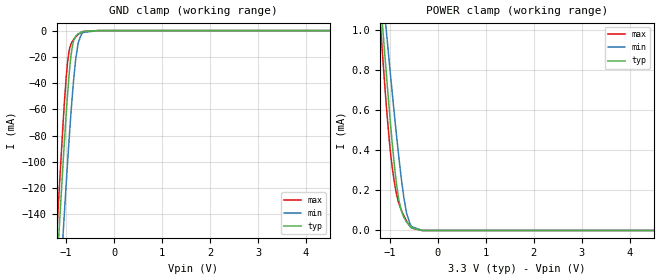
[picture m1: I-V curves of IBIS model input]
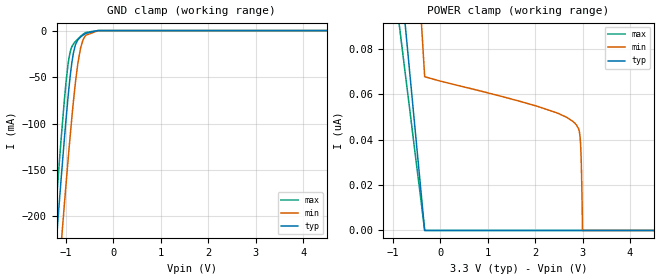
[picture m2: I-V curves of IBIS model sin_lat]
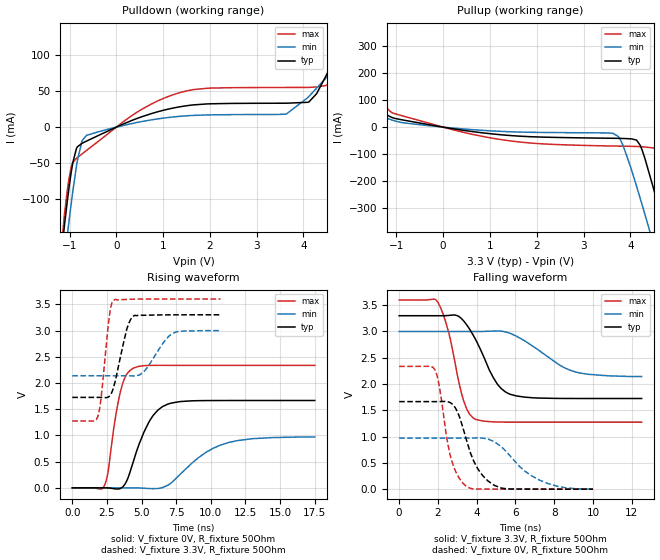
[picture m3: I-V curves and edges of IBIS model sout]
|Texas Instruments Incorporated
| 48 channels constant current LED driver with global brightness control,
| LED open-short detection and power save mode
| Marketing part#   Digital Voltage Range   Package-type   #pins
| TLC5954RTQR   3.0V-3.6V   QFN   56
| TLC5954RTQT   3.0V-3.6V   QFN   56
[IBIS Ver]   4.1
[File name]   tlc5954.ibs
[File Rev]   1.0
[Date]   2/19/2014
[Source]
| Texas Instruments Incorporated.
| Analog-eLab Design Center, HPA
| 12500 TI Blvd
| Dallas, TX -75243
[Notes]   Revision History:
| Rev 1.0: 2/19/2014
| - Initial version of the model
| - Model generated from simulations in TISPICE
| - Model matched to SPICE simulation
| - C_comp although listed in numerical order of value are
|   obtained from varying PVT conditions. For PVT conditions for
|   each specific value refer the buffer description under
|   respective [Model]. IBIS model user is responsible for using
|   appropriate C_comp to simulate for Signal Integrity.
[Disclaimer]
| This model is designed as an aid for customers of Texas Instruments.
| TI and its licensors and suppliers make no warranties, either expressed
| or implied, with respect to this  model, including the warranties of
| merchantability or fitness for a particular purpose. The model is
| provided solely on an "as is" basis. The entire risk as to its quality
| and performance is with the customer.
[Copyright]
(C) Copyright 2014 Texas Instruments Incorporated.All rights reserved.
|   TLC5954RTQ
[Component]   TLC5954RTQ
[Manufacturer]   TI
[Package]   |56 QFN   -  RTQ package
|   typ   min   max
R_pkg   0.01   0.008   0.12
L_pkg   1.0nH   0.8nH   1.2nH
C_pkg   0.2pF   0.16pF   0.24pF
[Pin]  signal_name   model_name   R_pin   L_pin   C_pin
1   GND   gnd   NA   NA   NA
2   OUTR14   nc   NA   NA   NA
3   OUTG14   nc   NA   NA   NA
4   OUTB14   nc   NA   NA   NA
5   OUTR15   nc   NA   NA   NA
6   OUTG15   nc   NA   NA   NA
7   OUTB15   nc   NA   NA   NA
8   OUTR0   nc   NA   NA   NA
9   OUTG0   nc   NA   NA   NA
10   OUTB0   nc   NA   NA   NA
11   OUTR1   nc   NA   NA   NA
12   OUTG1   nc   NA   NA   NA
13   OUTB1   nc   NA   NA   NA
14   OUTR2   nc   NA   NA   NA
15   OUTG2   nc   NA   NA   NA
16   OUTB2   nc   NA   NA   NA
17   OUTR3   nc   NA   NA   NA
18   OUTG3   nc   NA   NA   NA
19   OUTB3   nc   NA   NA   NA
20   OUTR4   nc   NA   NA   NA
21   OUTG4   nc   NA   NA   NA
22   OUTB4   nc   NA   NA   NA
23   OUTR5   nc   NA   NA   NA
24   OUTG5   nc   NA   NA   NA
25   OUTB5   nc   NA   NA   NA
26   SIN   sin_lat   NA   NA   NA
27   LAT   sin_lat   NA   NA   NA
28   SCLK   input   NA   NA   NA
29   BLANK   input   NA   NA   NA
30   OUTR6   nc   NA   NA   NA
31   OUTG6   nc   NA   NA   NA
32   OUTB6   nc   NA   NA   NA
33   OUTR7   nc   NA   NA   NA
34   OUTG7   nc   NA   NA   NA
35   OUTB7   nc   NA   NA   NA
36   OUTR8   nc   NA   NA   NA
37   OUTG8   nc   NA   NA   NA
38   OUTB8   nc   NA   NA   NA
39   OUTR9   nc   NA   NA   NA
40   OUTG9   nc   NA   NA   NA
41   OUTB9   nc   NA   NA   NA
42   SOUT   sout   NA   NA   NA
43   VCC   power   NA   NA   NA
44   OUTR10   nc   NA   NA   NA
45   OUTG10   nc   NA   NA   NA
46   OUTB10   nc   NA   NA   NA
47   OUTR11   nc   NA   NA   NA
48   OUTG11   nc   NA   NA   NA
49   OUTB11   nc   NA   NA   NA
50   OUTR12   nc   NA   NA   NA
51   OUTG12   nc   NA   NA   NA
52   OUTB12   nc   NA   NA   NA
53   OUTR13   nc   NA   NA   NA
54   OUTG13   nc   NA   NA   NA
55   OUTB13   nc   NA   NA   NA
56   GND   gnd   NA   NA   NA
| Models and submodels in the file (3): input (Input), sin_lat (Input), sout (Output)
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|   input Model
[Model]   input
Model_type   Input
Vinl = 0.99
Vinh = 2.31
|   typ   min   max
|   (nom PVT)   (fast PVT)   (slow PVT)
C_comp   6.057e-13   5.856e-13   6.288e-13
[Model spec]
|subparameter
Vinl   0.99   0.9   1.08
Vinh   2.31   2.1   2.52
| Where nom  PVT is Nominal Process, 3.3V, 27C
|   Fast PVT is Strong Process,  3.6V, -40C
|   Slow PVT is Weak Process,   3V, 125C
[Voltage Range]   3.3   3   3.6
|Junction Temperature
[Temperature Range]   27   125   -40
[Power Clamp Reference]   3.3   3   3.6
[GND Clamp Reference]   0   0   0
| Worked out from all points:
|   GND clamp passes 1 mA (typ) near -0.67 V on its own axis
|   POWER clamp passes 1 mA (typ) near -1.15 V on its own axis
[GND Clamp]
|   Voltage   I(typ)   I(min)   I(max)
-3.3V     -1.715A    -1.712A    -1.747A
-1.323V   -269.6mA   -320.3mA   -244.1mA
-1.169V   -166.8mA   -220.5mA   -137.4mA
-1.143V   -150.2mA   -204.2mA   -120.3mA
-1.059V   -98.17mA   -152.5mA   -67.79mA
-970.2mV  -48.9mA    -100.7mA   -24.26mA
-924mV    -28.13mA   -75.67mA   -13.15mA
-884.4mV  -15.24mA   -55.81mA   -9.19mA
-801mV    -4.374mA   -22.06mA   -4.837mA
-749.1mV  -2.498mA   -9.513mA   -2.927mA
-683.1mV  -1.186mA   -2.817mA   -1.271mA
6.6V      0A         0A         0A
[POWER Clamp]
|   Voltage   I(typ)   I(min)   I(max)
-3.3V     8.128mA    7.259mA    9.028mA
-1.263V   1.36mA     1.486mA    1.259mA
-1.176V   1.089mA    1.257mA    955uA
-1.146V   997.3uA    1.179mA    853.4uA
-1.072V   773.5uA    987.4uA    614.2uA
-956.4mV  449.2uA    698.7uA    324.4uA
-888mV    284.2uA    534.4uA    214uA
-822mV    165.2uA    384.2uA    142.4uA
-758.4mV  96.08uA    252.3uA    100.1uA
-654mV    42.86uA    88.7uA     47.46uA
-543mV    13.09uA    19.18uA    11.6uA
6.6V      0A         0A         0A
|   sin_lat Model
[Model]   sin_lat
Model_type   Input
Vinl = 0.99
Vinh = 2.31
|   typ   min   max
|   (nom PVT)   (fast PVT)   (slow PVT)
C_comp   1.585e-12   1.538e-12   1.659e-12
[Model spec]
|subparameter
Vinl   0.99   0.9   1.08
Vinh   2.31   2.1   2.52
| Where nom  PVT is Nominal Process, 3.3V, 27C
|   Fast PVT is Strong Process,  3.6V, -40C
|   Slow PVT is Weak Process,   3V, 125C
[Voltage Range]   3.3   3   3.6
|Junction Temperature
[Temperature Range]   27   125   -40
[Power Clamp Reference]   3.3   3   3.6
[GND Clamp Reference]   0   0   0
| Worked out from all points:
|   GND clamp passes 1 mA (typ) near -0.41 V on its own axis
[GND Clamp]
|   Voltage   I(typ)   I(min)   I(max)
-3.3V     -1.746A    -1.777A    -1.738A
-1.284V   -280.1mA   -349.1mA   -239.1mA
-1.144V   -186mA     -256.6mA   -143.3mA
-1.101V   -158.3mA   -229.1mA   -115.5mA
-1.039V   -119.3mA   -189.8mA   -77.38mA
-960mV    -73.11mA   -141.2mA   -37.54mA
-913.2mV  -49.56mA   -113.8mA   -23.26mA
-844.8mV  -24.36mA   -76.62mA   -14.51mA
-750mV    -9.939mA   -35.18mA   -8.982mA
-693mV    -6.943mA   -18.81mA   -6.242mA
-579mV    -2.905mA   -4.958mA   -1.961mA
6.6V      0A         0A         0A
[POWER Clamp]
|   Voltage   I(typ)   I(min)   I(max)
-3.3V     55.85uA    43.44uA    72.17uA
-1.224V   197.7nA    378.1nA    151.3nA
-330mV    0A         67.78nA    0A
2.043V    0A         54.76nA    0A
2.835V    0A         47.33nA    0A
2.916V    0A         44.78nA    0A
2.949V    0A         40.68nA    0A
2.964V    0A         34.93nA    0A
2.976V    0A         26.64nA    0A
2.991V    0A         10.47nA    0A
2.997V    0A         0A         0A
6.6V      0A         0A         0A
|   sout Model
[Model]   sout
Model_type   Output
Polarity   Non-Inverting
Vmeas = 1.65
Vref = 0
Cref = 15pF
Rref = 100
|   typ   min   max
|   (nom PVT)   (fast PVT)   (slow PVT)
C_comp   8.925e-13   8.663e-13   9.450e-13
| Where nom  PVT is Nominal Process, 3.3V, 27C
|   Fast PVT is Strong Process,  3.6V, -40C
|   Slow PVT is Weak Process,   3V, 125C
[Voltage Range]   3.3   3   3.6
|Junction Temperature
[Temperature Range]   27   125   -40
[Pullup Reference]   3.3   3   3.6
[Pulldown Reference]   0   0   0
[Power Clamp Reference]   3.3   3   3.6
[GND Clamp Reference]   0   0   0
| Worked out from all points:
|   slope of the pulldown table from 0 to 0.495 V, typ, clamps not added: 37.1 ohm
|   slope of the pullup table from 0 to 0.495 V, typ, clamps not added: 37.2 ohm
|   falling waveform, V_fixture 3.3V, R_fixture 50Ohm: 20-80 % time 1.26ns typ, 2.06ns min, 841ps max; typ from 3.3 V to 1.73 V
|   rising waveform, V_fixture 0V, R_fixture 50Ohm: 20-80 % time 1.51ns typ, 2.82ns min, 837ps max; typ from 0 V to 1.67 V
|   rising waveform, V_fixture 3.3V, R_fixture 50Ohm: 20-80 % time 792ps typ, 1.3ns min, 522ps max; typ from 1.73 V to 3.3 V
|   falling waveform, V_fixture 0V, R_fixture 50Ohm: 20-80 % time 1ns typ, 1.76ns min, 667ps max; typ from 1.67 V to 0 V
[Pulldown]
|   Voltage   I(typ)   I(min)   I(max)
-3.3V     -1.604A    -1.523A    -1.834A
-1.208V   -197.9mA   -241.7mA   -190.7mA
-1.049V   -104.3mA   -152mA     -89.41mA
-851.4mV  -29.68mA   -54.34mA   -43.44mA
-636mV    -19.43mA   -11.44mA   -32.43mA
1.254V    27.14mA    14.45mA    46.04mA
3.633V    33.37mA    18.22mA    55.34mA
4.115V    35.06mA    42.81mA    55.42mA
4.555V    81.29mA    73.9mA     61.03mA
4.779V    111.7mA    90.06mA    112.2mA
5.419V    199.6mA    136.4mA    301.4mA
6.6V      352.5mA    219.9mA    597.8mA
[Pullup]
|   Voltage   I(typ)   I(min)   I(max)
-3.3V     319.3mA    181.5mA    602mA
-2.396V   204.1mA    117.3mA    403.6mA
-1.054V   33.21mA    23.97mA    50.62mA
1.265V    -28.61mA   -15.95mA   -46.72mA
3.633V    -41.13mA   -23.24mA   -69.74mA
3.846V    -41.83mA   -68.56mA   -70.34mA
4.134V    -48.12mA   -218.9mA   -71.38mA
4.483V    -219.2mA   -424.7mA   -76.67mA
4.71V     -366.7mA   -562mA     -177.5mA
4.877V    -478.3mA   -664.4mA   -304.9mA
5.031V    -581.6mA   -758.7mA   -427.3mA
6.6V      -1.646A    -1.732A    -1.677A
[Ramp]
R_load = 50
|   typ   min   max
dV/dt_r   0.999443/1.50998e-09   0.582144/2.7836e-09   1.40136/8.33845e-10
dV/dt_f   0.945137/1.25907e-09   0.51741/2.07859e-09   1.39473/8.39673e-10
[Falling Waveform]
V_fixture = 3.3V
V_fixture_min = 3V
V_fixture_max = 3.6V
R_fixture = 50Ohm
|   Time   V(typ)   V(min)   V(max)
0s        3.3V       3V         3.6V
1.998ns   3.3V       3V         3.556V
2.578ns   3.306V     3V         2.947V
3.334ns   3.198V     3V         1.674V
3.612ns   3.057V     3V         1.44V
3.966ns   2.831V     3V         1.325V
5.048ns   2.009V     3.009V     1.278V
5.714ns   1.806V     2.966V     1.275V
9.056ns   1.725V     2.234V     1.275V
12.51ns   1.725V     2.143V     1.275V
[Rising Waveform]
V_fixture = 0V
V_fixture_min = 0V
V_fixture_max = 0V
R_fixture = 50Ohm
|   Time   V(typ)   V(min)   V(max)
0s        1.217nV    7.604nV    889.5pV
2.3ns     373.7uV    651.9nV    30.77mV
2.58ns    -1.087mV   684.4nV    297mV
3.056ns   -17.87mV   -4.722uV   1.243V
3.484ns   -11.65mV   -15.76uV   1.844V
4.394ns   487.9mV    286.8uV    2.281V
5.664ns   1.312V     -13.94mV   2.336V
6.978ns   1.603V     62.95mV    2.336V
10.69ns   1.665V     813.6mV    2.336V
17.51ns   1.666V     970.2mV    2.336V
[Rising Waveform]
V_fixture = 3.3V
V_fixture_min = 3V
V_fixture_max = 3.6V
R_fixture = 50Ohm
|   Time   V(typ)   V(min)   V(max)
0s        1.725V     2.138V     1.276V
1.852ns   1.725V     2.138V     1.366V
2.092ns   1.725V     2.138V     1.741V
2.646ns   1.739V     2.138V     3.205V
2.934ns   1.877V     2.138V     3.562V
3.904ns   2.993V     2.137V     3.594V
4.348ns   3.262V     2.135V     3.598V
5.22ns    3.291V     2.23V      3.6V
7.358ns   3.299V     2.959V     3.6V
10.71ns   3.3V       2.998V     3.6V
[Falling Waveform]
V_fixture = 0V
V_fixture_min = 0V
V_fixture_max = 0V
R_fixture = 50Ohm
|   Time   V(typ)   V(min)   V(max)
0s        1.666V     970.6mV    2.336V
1.85ns    1.665V     970.6mV    2.267V
2.076ns   1.666V     970.6mV    1.949V
2.696ns   1.632V     970.6mV    559.2mV
3.082ns   1.402V     970.4mV    218.4mV
3.522ns   872.8mV    971mV      40.8mV
4.164ns   327.6mV    975.4mV    2.758mV
5.262ns   22.37mV    810.3mV    279.7uV
7.236ns   891.6uV    172.3mV    19.1uV
9.999ns   114.5uV    3.619mV    8.213uV
